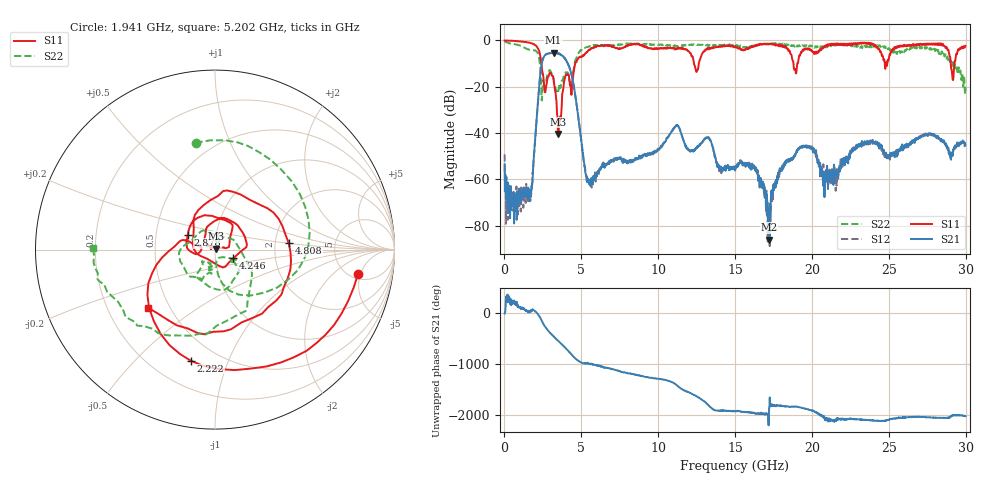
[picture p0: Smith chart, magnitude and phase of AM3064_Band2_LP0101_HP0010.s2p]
# Hz S DB R 50.0
!freq dBS11 angS11 dBS21 angS21 dBS12 angS12 dBS22 angS22
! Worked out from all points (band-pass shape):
!   1600 points, 10 MHz to 29.98 GHz, reference 50 ohm
!   highest |S21| = -5.32 dB at 3.196 GHz (marker M1); lowest = -85.9 dB at 17.2 GHz (marker M2)
!   |S21| within 3 dB of the highest: 2.486 GHz to 3.973 GHz (1.488 GHz wide, 46.1 % of centre)
!   lowest |S11| = -40.4 dB at 3.478 GHz (marker M3), VSWR 1.02, Z = 50.8 + j0.587 ohm
!   |S11| at or under -10 dB: 2.401 GHz to 4.594 GHz (2.194 GHz wide, 62.7 % of centre); 12.33 GHz to 12.64 GHz (312.4 MHz wide, 2.5 % of centre); 18.8 GHz to 19.05 GHz (250.1 MHz wide, 1.32 % of centre)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
!   |S22| runs from -25.9 to -0.3 dB; largest |S21 - S12| = 0.018
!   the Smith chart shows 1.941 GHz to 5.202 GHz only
!   S11 on the Smith chart (normalised r, x): 1.941 GHz: 5.82, -4.55; 2.222 GHz: 0.36, -0.74; 2.878 GHz: 0.73, +0.12; 4.246 GHz: 1.22, -0.12; 4.808 GHz: 2.38, +0.21; 5.202 GHz: 0.38, -0.33
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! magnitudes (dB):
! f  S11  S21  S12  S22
! 10 MHz  0.0  -53.4  -49.2  -0.3
! 722.3 MHz  -0.2  -71.4  -65.9  -1.7
! 1.659 GHz  -1.1  -67.0  -66.3  -4.2
! 1.941 GHz  -1.8  -47.9  -48.3  -4.4
! 2.222 GHz  -4.0  -23.0  -22.9  -6.4
! 2.878 GHz  -15.3  -5.6  -5.6  -13.5
! 3.196 GHz  -16.9  -5.3  -5.3  -16.7
! 3.478 GHz  -40.4  -5.6  -5.7  -21.3
! 4.246 GHz  -18.9  -12.0  -12.0  -17.8
! 4.808 GHz  -7.7  -33.3  -33.2  -5.6
! 5.015 GHz  -7.3  -44.3  -43.8  -4.2
! 5.202 GHz  -6.1  -54.4  -54.2  -3.3
! 10 GHz  -3.5  -47.3  -47.2  -1.9
! 11.22 GHz  -3.8  -36.5  -36.6  -2.4
! 15 GHz  -2.6  -56.1  -55.7  -2.0
! 16.34 GHz  -2.3  -56.4  -55.5  -2.4
! 17.2 GHz  -1.5  -85.9  -84.8  -1.6
! 18.21 GHz  -2.5  -53.6  -53.6  -1.7
! 19.99 GHz  -4.3  -46.9  -45.7  -2.2
! 20.82 GHz  -2.7  -67.6  -60.1  -2.5
! 25 GHz  -8.0  -49.8  -50.0  -3.3
! 29.98 GHz  -2.4  -45.2  -45.3  -20.2
